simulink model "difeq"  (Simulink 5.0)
settings: Solver=ode45  StartTime=0.0  StopTime=200  RelTol=1e-6
libraries: simulink x7

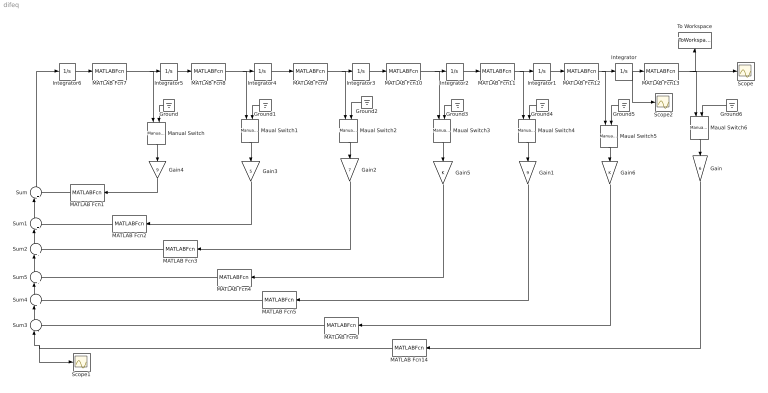
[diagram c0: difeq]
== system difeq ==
  Gain : Gain  Orientation=down  Gain=6
  Gain1 : Gain  Orientation=down  Gain=9
  Gain2 : Gain  Orientation=down  Gain=7
  Gain3 : Gain  Orientation=down  Gain=5
  Gain4 : Gain  Orientation=down  Gain=9
  Gain5 : Gain  Orientation=down
  Gain6 : Gain  Orientation=down
  Ground{,1..6} (7 alike) : Ground  Orientation=left
  Integrator : Integrator  InitialCondition=1
  Integrator{1..6} (6 alike) : Integrator
  MATLAB Fcn{1..6,14} (7 alike) : MATLABFcn  Orientation=left  MATLABFcn=satamp
  MATLAB Fcn{7..13} (7 alike) : MATLABFcn  MATLABFcn=satamp
  Manual Switch : simulink/Signal Routing/Manual Switch  Orientation=down  sw=1  action=0
  Maual Switch{1..2,4,6} (4 alike) : simulink/Signal Routing/Manual Switch  Orientation=down  sw=1  action=0
  Maual Switch3 : simulink/Signal Routing/Manual Switch  Orientation=down  sw=0  action=0
  Maual Switch5 : simulink/Signal Routing/Manual Switch  Orientation=down  sw=0  action=0
  Scope : Scope
  Scope1 : Scope
  Scope2 : Scope
  Sum{,1..2,4..5} (5 alike) : Sum  Orientation=up  Inputs=|+-
  Sum3 : Sum  Orientation=up  Inputs=|--
  To Workspace : ToWorkspace  VariableName=y  SampleTime=-1  SaveFormat=Array
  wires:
  Integrator/1 -> MATLAB Fcn13/1, Scope2/1
  Integrator1/1 -> MATLAB Fcn12/1
  Integrator2/1 -> MATLAB Fcn11/1
  Integrator3/1 -> MATLAB Fcn10/1
  Integrator4/1 -> MATLAB Fcn9/1
  Integrator5/1 -> MATLAB Fcn8/1
  Integrator6/1 -> MATLAB Fcn7/1
  Sum/1 -> Integrator6/1
  Sum1/1 -> Sum/1
  Sum2/1 -> Sum1/1
  Sum3/1 -> Sum4/1
  Sum5/1 -> Sum2/1
  Sum4/1 -> Sum5/1
  Ground/1 -> Manual Switch/2
  Ground6/1 -> Maual Switch6/2
  Ground5/1 -> Maual Switch5/2
  Ground4/1 -> Maual Switch4/2
  Ground3/1 -> Maual Switch3/2
  Ground2/1 -> Maual Switch2/2
  Ground1/1 -> Maual Switch1/2
  MATLAB Fcn7/1 -> Integrator5/1, Manual Switch/1
  MATLAB Fcn8/1 -> Integrator4/1, Maual Switch1/1
  MATLAB Fcn9/1 -> Integrator3/1, Maual Switch2/1
  MATLAB Fcn10/1 -> Integrator2/1, Maual Switch3/1
  MATLAB Fcn11/1 -> Integrator1/1, Maual Switch4/1
  MATLAB Fcn12/1 -> Integrator/1, Maual Switch5/1
  MATLAB Fcn13/1 -> Scope/1, To Workspace/1, Maual Switch6/1
  Manual Switch/1 -> Gain4/1
  Maual Switch1/1 -> Gain3/1
  Maual Switch2/1 -> Gain2/1
  Maual Switch3/1 -> Gain5/1
  Maual Switch4/1 -> Gain1/1
  Maual Switch5/1 -> Gain6/1
  Maual Switch6/1 -> Gain/1
  Gain4/1 -> MATLAB Fcn1/1
  Gain3/1 -> MATLAB Fcn2/1
  Gain2/1 -> MATLAB Fcn3/1
  Gain5/1 -> MATLAB Fcn4/1
  Gain1/1 -> MATLAB Fcn5/1
  Gain/1 -> MATLAB Fcn14/1
  Gain6/1 -> MATLAB Fcn6/1
  MATLAB Fcn1/1 -> Sum/2
  MATLAB Fcn2/1 -> Sum1/2
  MATLAB Fcn3/1 -> Sum2/2
  MATLAB Fcn4/1 -> Sum5/2
  MATLAB Fcn5/1 -> Sum4/2
  MATLAB Fcn6/1 -> Sum3/2
  MATLAB Fcn14/1 -> Sum3/1, Scope1/1
